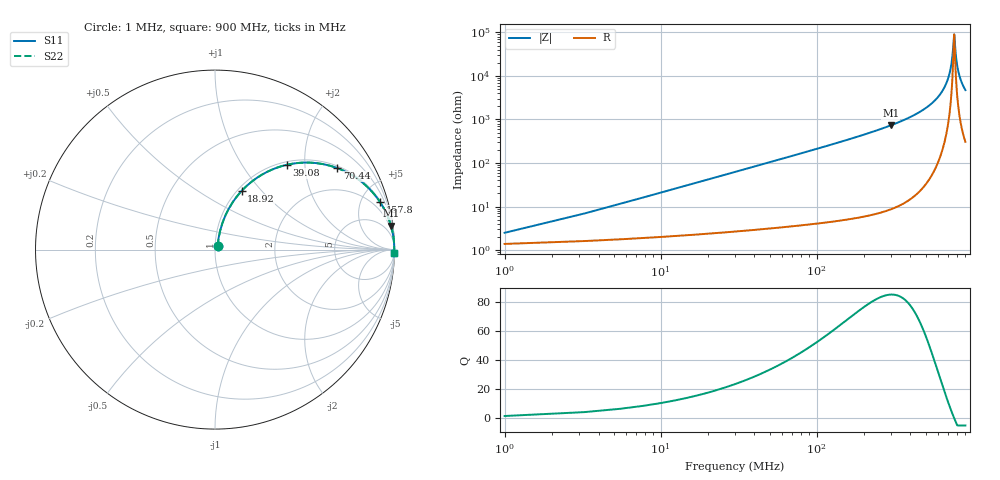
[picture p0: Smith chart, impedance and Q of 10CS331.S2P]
! Coilcraft 1008CS-331 Chip Inductor
! 02 July 2002
# MHZ S MA R 50
!Freq  MagS11  AngS11  MagS21  AngS21  MagS12  AngS12  MagS22  AngS22
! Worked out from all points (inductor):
!   403 points, 1 MHz to 900 MHz, reference 50 ohm
!   read as one part in series: L = 330 nH near 5.48 MHz
!   highest Q = 85 at 298.9 MHz (marker M1), where L = 390 nH
!   self-resonance near 762.6 MHz
!   S11 on the Smith chart (normalised r, x): 1 MHz: 1.03, +0.04; 18.92 MHz: 1.05, +0.79; 39.08 MHz: 1.06, +1.62; 70.44 MHz: 1.07, +2.95; 157.8 MHz: 1.10, +6.84; 900 MHz: 7, -95
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1  0.02458 55.1  0.9861 -1.2  0.9861 -1.2  0.02458 55.1
9.96  0.1994 73.0  0.9609 -11.4  0.9609 -11.4  0.1994 73.0
18.92  0.3588 65.6  0.9124 -21.0  0.9124 -21.0  0.3588 65.6
39.08  0.6201 49.7  0.7628 -38.3  0.7628 -38.3  0.6201 49.7
70.44  0.8184 33.7  0.5554 -54.9  0.5554 -54.9  0.8184 33.7
104.04  0.9039 24.3  0.4111 -64.7  0.4111 -64.7  0.9039 24.3
151.08  0.952 17.0  0.292 -72.2  0.292 -72.2  0.952 17.0
157.8  0.956 16.2  0.2796 -72.9  0.2796 -72.9  0.956 16.2
298.92  0.9892 7.8  0.1351 -81.6  0.1351 -81.6  0.9892 7.8
301.16  0.9894 7.7  0.1337 -81.6  0.1337 -81.6  0.9894 7.7
451.24  0.9966 4.0  0.06922 -85.2  0.06922 -85.2  0.9966 4.0
601.32  0.9986 1.7  0.03031 -86.5  0.03031 -86.5  0.9986 1.7
661.8  0.9988 1.0  0.018 -85.8  0.018 -85.8  0.9988 1.0
704.36  0.9989 0.6  0.0101 -83.5  0.0101 -83.5  0.9989 0.6
733.48  0.9989 0.3  0.005037 -77.4  0.005037 -77.4  0.9989 0.3
751.4  0.9989 0.1  0.002169 -59.5  0.002169 -59.5  0.9989 0.1
760.36  0.9989 0.0  0.00117 -18.6  0.00117 -18.6  0.9989 0.0
764.84  0.9989 -0.0  0.001175 18.2  0.001175 18.2  0.9989 -0.0
785  0.9988 -0.2  0.00383 72.4  0.00383 72.4  0.9988 -0.2
809.64  0.9988 -0.4  0.007654 80.6  0.007654 80.6  0.9988 -0.4
847.72  0.9987 -0.8  0.01344 83.9  0.01344 83.9  0.9987 -0.8
900  0.9984 -1.2  0.02105 85.1  0.02105 85.1  0.9984 -1.2
